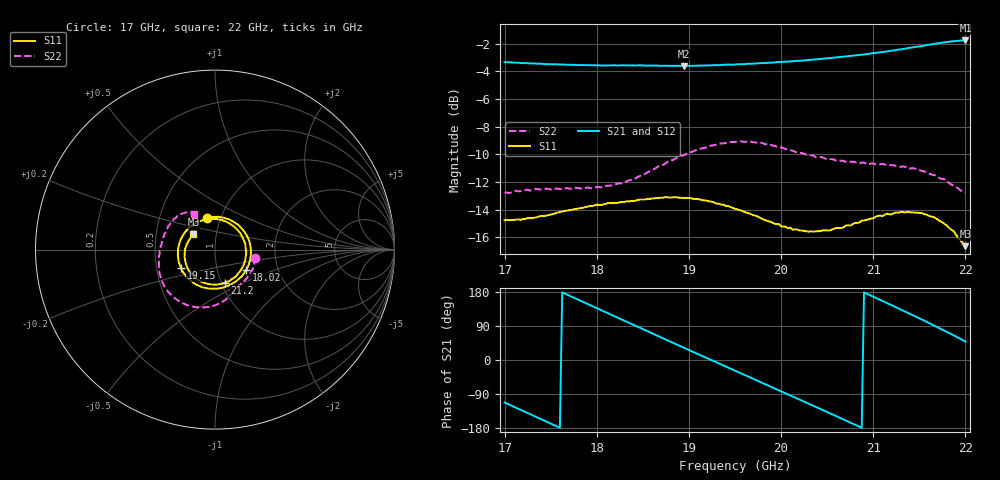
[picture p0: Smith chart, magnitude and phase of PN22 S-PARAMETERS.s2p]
!Agilent Technologies,N5230C,MY49001096,A.09.42.22
!Agilent N5230C: A.09.42.22
!Date: Monday, February 23, 2015 19:26:24
!Correction: S11(Full 2 Port(1,2))
!S21(Full 2 Port(1,2))
!S12(Full 2 Port(1,2))
!S22(Full 2 Port(1,2))
!S2P File: Measurements: S11, S21, S12, S22:
# Hz S  dB  R 50
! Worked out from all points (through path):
!   201 points, 17 GHz to 22 GHz, reference 50 ohm
!   highest |S21| = -1.75 dB at 22 GHz (marker M1); lowest = -3.6 dB at 18.95 GHz (marker M2)
!   group delay of S21, straight-line fit = 307 ps
!   lowest |S11| = -16.7 dB at 22 GHz (marker M3), VSWR 1.34, Z = 38.7 + j6.69 ohm
!   |S11| at or under -10 dB: start of sweep to end of sweep
!   |S22| runs from -12.8 to -9.1 dB; largest |S21 - S12| = 0.0027
!   S11 on the Smith chart (normalised r, x): 17 GHz: 0.86, +0.32; 18.02 GHz: 1.38, -0.33; 19.15 GHz: 0.67, -0.15; 21.2 GHz: 1.04, -0.40; 22 GHz: 0.77, +0.13
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1.7e10  -14.78 103.7  -3.33 -112.2  -3.32 -112.2  -12.80 -11.2
1.7425e10  -14.48 41.5  -3.46 -159.5  -3.45 -159.5  -12.50 -31.4
1.7625e10  -14.13 15.0  -3.49 178.3  -3.49 178.3  -12.50 -40.0
1.785e10  -13.88 -13.2  -3.54 153.3  -3.54 153.4  -12.44 -48.9
1.8025e10  -13.65 -33.0  -3.55 134.1  -3.55 134.0  -12.36 -54.6
1.8375e10  -13.38 -70.4  -3.56 95.2  -3.54 95.2  -11.85 -66.2
1.8675e10  -13.15 -100.6  -3.58 61.9  -3.59 61.9  -10.85 -78.2
1.895e10  -13.18 -129.6  -3.60 31.8  -3.59 31.8  -10.04 -92.8
1.915e10  -13.33 -151.1  -3.58 10.0  -3.57 9.9  -9.56 -104.6
1.95e10  -13.94 169.0  -3.49 -28.1  -3.48 -28.1  -9.11 -126.6
1.995e10  -15.06 109.9  -3.33 -77.1  -3.34 -77.2  -9.43 -154.5
2.015e10  -15.43 80.3  -3.24 -99.0  -3.24 -99.0  -9.81 -164.9
2.035e10  -15.60 49.4  -3.13 -120.9  -3.14 -121.0  -10.09 -174.2
2.06e10  -15.33 11.1  -2.98 -148.3  -2.99 -148.4  -10.47 174.9
2.08e10  -14.96 -18.7  -2.84 -170.4  -2.85 -170.5  -10.55 166.8
2.1e10  -14.63 -46.5  -2.66 167.2  -2.67 167.2  -10.66 158.1
2.1175e10  -14.36 -70.2  -2.52 147.5  -2.51 147.5  -10.79 150.4
2.12e10  -14.34 -73.5  -2.49 144.6  -2.47 144.6  -10.78 149.3
2.1425e10  -14.20 -104.3  -2.25 118.8  -2.25 118.7  -11.00 139.0
2.1625e10  -14.51 -134.8  -2.05 95.3  -2.04 95.2  -11.45 130.4
2.1825e10  -15.35 -171.4  -1.84 71.0  -1.83 70.9  -12.08 123.3
2.2e10  -16.65 145.0  -1.75 48.6  -1.75 48.6  -12.75 120.8
